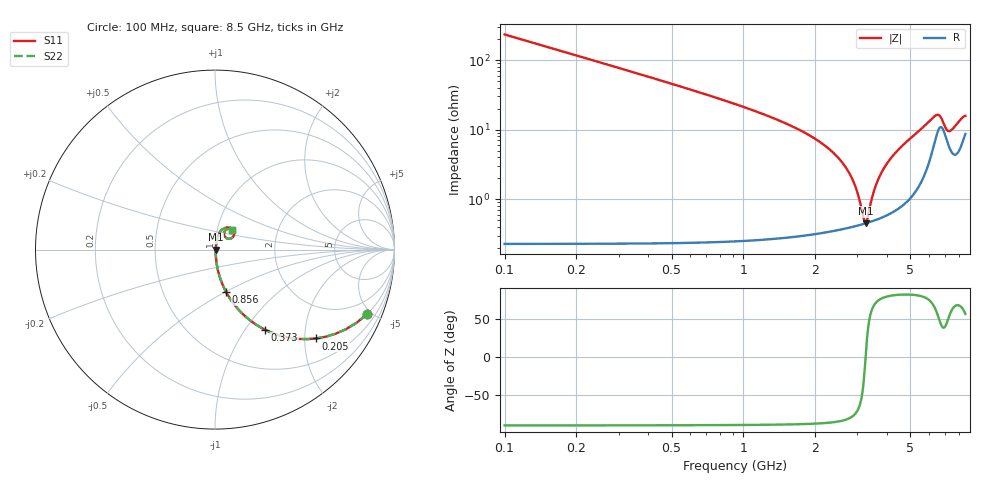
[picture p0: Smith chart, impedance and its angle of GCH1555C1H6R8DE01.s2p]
!Murata Part Number: GCH1555C1H6R8DE01
!These Parameters are Measured in Series Mode Connection
!Data Generated on Mar 13, 2026
!  o--ll--o
!Port1  Port2
!  o------o
!Operation Temp=25[degC], DC Bias Voltage=0[V]
!Freq. Start=100[MHz] Stop=9[GHz] 401[Steps]
# Hz S RI R 50
!Freq.(Hz) S11(Real) S11(Imag) S21(Real) S21(Imag) S12(Real) S12(Imag) S22(Real) S22(Imag)
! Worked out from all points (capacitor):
!   401 points, 100 MHz to 8.5 GHz, reference 50 ohm
!   read as one part in series: C = 6.8 pF near 142 MHz
!   lowest |Z| = 449 mohm at 3.25 GHz (marker M1)
!   series resonance near 3.248 GHz, so ESL is about 350 pH
!   S11 on the Smith chart (normalised r, x): 100 MHz: 1.00, -4.68; 205 MHz: 1.00, -2.27; 373 MHz: 1.00, -1.24; 856 MHz: 1.00, -0.51; 8.5 GHz: 1.17, +0.26
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1e8  0.8451 -0.3613  0.1549 0.3613  0.1549 0.3613  0.8451 -0.3613
2.05e8  0.5638 -0.4949  0.4362 0.4949  0.4362 0.4949  0.5638 -0.4949
3.73e8  0.278 -0.4462  0.722 0.4462  0.722 0.4462  0.278 -0.4462
5.62e8  0.1419 -0.3461  0.8581 0.3461  0.8581 0.3461  0.1419 -0.3461
8.56e8  0.063 -0.2382  0.937 0.2382  0.937 0.2382  0.063 -0.2382
1.507e9  0.0175 -0.1201  0.9825 0.1201  0.9825 0.1201  0.0175 -0.1201
2.431e9  0.00535 -0.0427  0.9946 0.0427  0.9946 0.0427  0.00535 -0.0427
2.704e9  0.00453 -0.027  0.9955 0.027  0.9955 0.027  0.00453 -0.027
2.914e9  0.00429 -0.016  0.9957 0.016  0.9957 0.016  0.00429 -0.016
3.04e9  0.00428 -0.00976  0.9957 0.00976  0.9957 0.00976  0.00428 -0.00976
3.187e9  0.00439 -0.00279  0.9956 0.00279  0.9956 0.00279  0.00439 -0.00279
3.25e9  0.00447 0.000106  0.9955 -0.000106  0.9955 -0.000106  0.00447 0.000106
3.292e9  0.00453 0.00201  0.9955 -0.00201  0.9955 -0.00201  0.00453 0.00201
3.502e9  0.00498 0.0113  0.995 -0.0113  0.995 -0.0113  0.00498 0.0113
3.67e9  0.00549 0.0184  0.9945 -0.0184  0.9945 -0.0184  0.00549 0.0184
3.943e9  0.0066 0.0297  0.9934 -0.0297  0.9934 -0.0297  0.0066 0.0297
4.3e9  0.00864 0.044  0.9914 -0.044  0.9914 -0.044  0.00864 0.044
5.707e9  0.0323 0.1039  0.9677 -0.1039  0.9677 -0.1039  0.0323 0.1039
6.505e9  0.0985 0.1112  0.9015 -0.1112  0.9015 -0.1112  0.0985 0.1112
7.114e9  0.0689 0.0614  0.9311 -0.0614  0.9311 -0.0614  0.0689 0.0614
7.366e9  0.054 0.0741  0.946 -0.0741  0.946 -0.0741  0.054 0.0741
8.5e9  0.0934 0.1103  0.9066 -0.1103  0.9066 -0.1103  0.0934 0.1103
